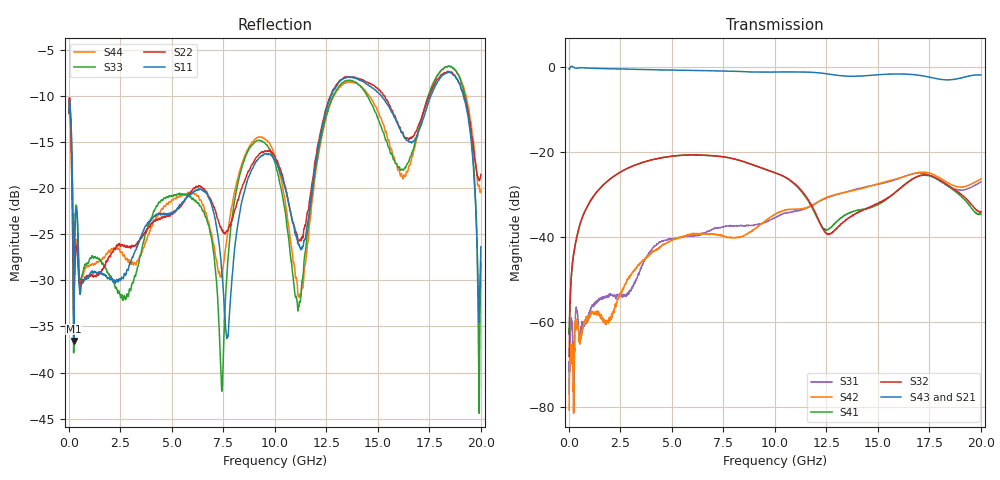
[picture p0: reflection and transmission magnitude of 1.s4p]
!Keysight Technologies,N5225A,MY51451420,A.10.40.12
!Date: Tuesday, October 13, 2015 10:29:25
!Correction: S11(Full 4 Port(1,2,3,4))
!S12(Full 4 Port(1,2,3,4))
!S13(Full 4 Port(1,2,3,4))
!S14(Full 4 Port(1,2,3,4))
!S21(Full 4 Port(1,2,3,4))
!S22(Full 4 Port(1,2,3,4))
!S23(Full 4 Port(1,2,3,4))
!S24(Full 4 Port(1,2,3,4))
!S31(Full 4 Port(1,2,3,4))
!S32(Full 4 Port(1,2,3,4))
!S33(Full 4 Port(1,2,3,4))
!S34(Full 4 Port(1,2,3,4))
!S41(Full 4 Port(1,2,3,4))
!S42(Full 4 Port(1,2,3,4))
!S43(Full 4 Port(1,2,3,4))
!S44(Full 4 Port(1,2,3,4))
!S4P File: Measurements: <S11,S12,S13,S14>,
!<S21,S22,S23,S24>,
!<S31,S32,S33,S34>,
!<S41,S42,S43,S44>:
# Hz S  dB  R 50
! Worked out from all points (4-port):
!   1999 points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, 20 MHz to 20 GHz, reference 50 ohm
!   strongest paths, dB at 20 MHz, 5.01 GHz, 10.01 GHz, 15.01 GHz, 20 GHz:
!     S43: -0.5, -0.8, -1.2, -1.9, -1.9
!     S21: -0.5, -0.8, -1.3, -2.2, -2.0
!     S32: -68.0, -21.0, -24.9, -32.0, -34.0
!     S41: -61.5, -21.0, -24.9, -32.4, -34.6
!     S42: -80.7, -40.7, -34.6, -27.5, -26.4
!     S31: -76.9, -40.5, -35.5, -27.6, -27.0
!   lowest |S11| = -36.6 dB at 240 MHz (marker M1), VSWR 1.03, Z = 50.2 - j1.47 ohm
!   |S11| at or under -10 dB: start of sweep to 12.74 GHz; 15.17 GHz to 17.58 GHz (2.411 GHz wide, 14.7 % of centre); 19.15 GHz to end of sweep
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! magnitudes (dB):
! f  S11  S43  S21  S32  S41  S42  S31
! 20 MHz  -11.8  -0.5  -0.5  -68.0  -61.5  -80.7  -76.9
! 240 MHz  -36.6  -0.1  -0.1  -44.1  -43.8  -81.4  -81.1
! 7.43 GHz  -28.9  -1.0  -1.0  -21.1  -21.1  -39.7  -37.7
! 8.83 GHz  -18.3  -1.2  -1.2  -22.8  -22.9  -38.8  -37.3
! 11.16 GHz  -26.2  -1.2  -1.3  -28.4  -28.5  -33.4  -33.7
! 18.49 GHz  -7.5  -3.1  -2.9  -28.1  -28.3  -27.5  -28.2
! 20 GHz  -26.4  -1.9  -2.0  -34.0  -34.6  -26.4  -27.0
